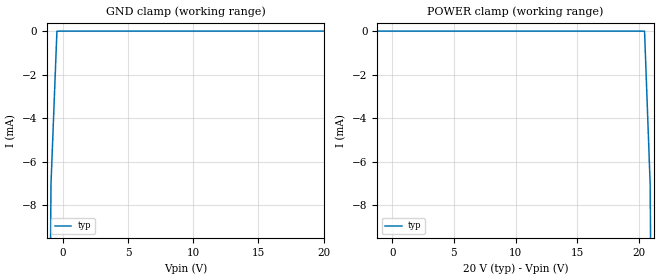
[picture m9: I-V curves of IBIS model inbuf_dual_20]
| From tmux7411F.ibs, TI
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| inbuf_dual_20
[Model]   inbuf_dual_20
Model_type   Input
Vinl = 1.3
Vinh = 0.8
|   typ   min   max
C_comp   1.598234e-12   NA   NA
[Voltage Range]   20   NA   NA
[Temperature Range]   27   NA   NA
[Power Clamp Reference]   20   NA   NA
[GND Clamp Reference]   0   NA   NA
[GND Clamp]
|   Voltage   I(typ)   I(min)   I(max)
-25V      -2.193A    NA         NA
-1.364V   -43.51mA   NA         NA
-909.1mV  -7.032mA   NA         NA
-454.5mV  -3.667uA   NA         NA
20V       1.067uA    NA         NA
[POWER Clamp]
|   Voltage   I(typ)   I(min)   I(max)
-5V       1.519uA    NA         NA
20.45V    -3.667uA   NA         NA
20.91V    -7.032mA   NA         NA
21.36V    -43.51mA   NA         NA
40V       -1.736A    NA         NA
